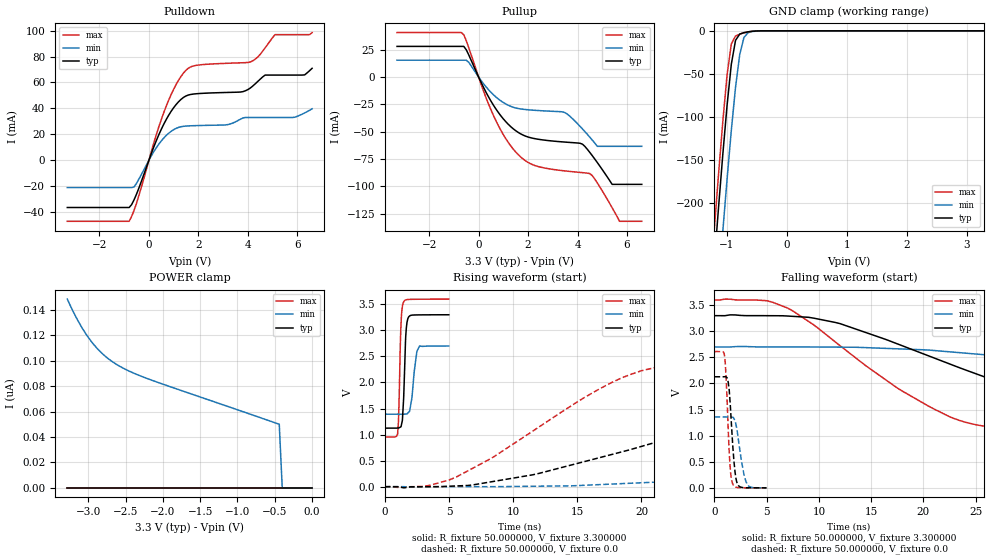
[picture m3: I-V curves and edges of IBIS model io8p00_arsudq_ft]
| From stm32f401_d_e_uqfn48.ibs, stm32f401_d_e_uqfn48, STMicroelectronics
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|   Model io8p00_arsudq_ft
[Model]  io8p00_arsudq_ft
Model_type I/O
Polarity   Non-Inverting
Enable   Active-Low
Vinl =   0.990000V
Vinh =   2.310000V
Vmeas =  1.650000V
Cref =   50.000000pF
Rref =   100.000000M
Vref =   0.0V
C_comp   2.292100pF   2.228000pF   2.366600pF
[Temperature Range]   25.000000   0.125000k   -40.000000
[Pullup Reference]   3.300000V   2.700000V   3.600000V
[Pulldown Reference]   0.0V   0.0V   0.0V
[POWER Clamp Reference]   3.300000V   2.700000V   3.600000V
[GND Clamp Reference]   0.0V   0.0V   0.0V
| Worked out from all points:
|   slope of the pulldown table from 0 to 0.495 V, typ, clamps not added: 20.9 ohm
|   slope of the pullup table from 0 to 0.495 V, typ, clamps not added: 22.6 ohm
|   GND clamp passes 1 mA (typ) near -0.62 V on its own axis
|   rising waveform, R_fixture 50.000000, V_fixture 3.300000: 20-80 % time 190ps typ, 338ps min, 164ps max; typ from 1.12 V to 3.3 V
|   rising waveform, R_fixture 50.000000, V_fixture 0.0: 20-80 % time 19.7ns typ, 51ns min, 10.3ns max; typ from 0 V to 2.13 V
|   falling waveform, R_fixture 50.000000, V_fixture 3.300000: 20-80 % time 18.6ns typ, 39.1ns min, 11.5ns max; typ from 3.3 V to 1.12 V
|   falling waveform, R_fixture 50.000000, V_fixture 0.0: 20-80 % time 434ps typ, 633ps min, 343ps max; typ from 2.13 V to 0 V
[Pulldown]
|Voltage   I(typ)   I(min)   I(max)
-3.3V     -36.46mA   -21.09mA   -47.09mA
-800mV    -36.46mA   -21.09mA   -47.09mA
-600mV    -30.5mA    -20.54mA   -38.69mA
700mV     31.4mA     19.11mA    41.71mA
1.2V      45.15mA    25.37mA    61.75mA
1.6V      50.35mA    26.5mA     71.06mA
3.1V      52.28mA    27.26mA    74.76mA
4.1V      55.7mA     32.99mA    75.81mA
4.7V      65.72mA    32.99mA    86.7mA
5.1V      65.72mA    32.99mA    96.91mA
6.3V      65.88mA    36.51mA    96.91mA
6.6V      70.94mA    39.72mA    98.51mA
[Pullup]
|Voltage   I(typ)   I(min)   I(max)
-3.3V     28.04mA    15.43mA    40.69mA
-700mV    28.04mA    15.43mA    40.69mA
-400mV    20.31mA    13.47mA    26.93mA
600mV     -25.77mA   -16.23mA   -35.14mA
1.6V      -50.64mA   -28.81mA   -70.96mA
3.5V      -59.53mA   -32.65mA   -85.92mA
4.2V      -61.43mA   -47.48mA   -87.46mA
4.5V      -69.07mA   -55.12mA   -88.38mA
4.8V      -78.22mA   -63.4mA    -96.83mA
5.4V      -98.2mA    -63.4mA    -119.6mA
5.7V      -98.2mA    -63.4mA    -132mA
6.6V      -98.2mA    -63.4mA    -132mA
[GND_clamp]
|Voltage   I(typ)   I(min)   I(max)
-3.3V     -2.319A    -2.398A    -2.292A
-1.2V     -265.5mA   -356.1mA   -227.2mA
-1.13V    -202.6mA   -292.9mA   -164.1mA
-1.06V    -142.2mA   -231.2mA   -104.1mA
-990mV    -85.98mA   -171.6mA   -50.72mA
-920mV    -38.8mA    -115.5mA   -15.28mA
-850mV    -11.08mA   -65.6mA    -6.001mA
-780mV    -3.782mA   -27.42mA   -3.876mA
-710mV    -2.086mA   -7.69mA    -2.381mA
-640mV    -1.147mA   -2.118mA   -1.22mA
-570mV    -523.9uA   -798.4uA   -476.8uA
3.28V     0A         0A         0A
[POWER_clamp]
|Voltage   I(typ)   I(min)   I(max)
-3.28V    0A         148.5nA    0A
-3.2V     0A         138.6nA    0A
-3.12V    0A         129.7nA    0A
-3.04V    0A         122nA      0A
-2.96V    0A         115.3nA    0A
-2.8V     0A         105.1nA    0A
-2.6V     0A         96.44nA    0A
-2.4V     0A         90.52nA    0A
-2.16V    0A         84.97nA    0A
-440mV    0A         50.04nA    0A
-400mV    0A         0A         0A
0V        0A         0A         0A
[Ramp]
| variable   typ   min   max
dV/dt_r  1.27740/19.68906n   0.81540/50.98348n   1.56732/10.32996n
dV/dt_f  1.30734/18.58362n   0.78450/39.11759n   1.58789/11.43308n
R_load = 50.000000
[Rising Waveform]
R_fixture= 50.000000
V_fixture= 3.300000
V_fixture_min= 2.700000
V_fixture_max= 3.600000
|time   V(typ)   V(min)   V(max)
0s        1.124V     1.392V     953.5mV
1.001ns   1.126V     1.392V     1.018V
1.071ns   1.128V     1.392V     1.288V
1.251ns   1.149V     1.392V     3.035V
1.461ns   1.66V      1.391V     3.543V
1.632ns   2.882V     1.394V     3.586V
1.862ns   3.259V     1.43V      3.594V
2.503ns   3.297V     2.597V     3.597V
2.703ns   3.297V     2.698V     3.598V
4.985ns   3.3V       2.7V       3.6V
[Rising Waveform]
R_fixture= 50.000000
V_fixture= 0.0
V_fixture_min= 0.0
V_fixture_max= 0.0
|time   V(typ)   V(min)   V(max)
0s        4.932nV    245.7nV    3.133nV
5.506ns   13.81mV    -141.5uV   177.7mV
11.51ns   227.5mV    8.254mV    1.064V
19.02ns   703.8mV    64.87mV    2.142V
27.53ns   1.299V     163.4mV    2.488V
38.54ns   1.854V     360.2mV    2.577V
57.56ns   2.068V     710.1mV    2.608V
89.09ns   2.119V     1.139V     2.612V
117.6ns   2.128V     1.298V     2.612V
249.2ns   2.129V     1.359V     2.612V
[Falling Waveform]
R_fixture= 50.000000
V_fixture= 3.300000
V_fixture_min= 2.700000
V_fixture_max= 3.600000
|time   V(typ)   V(min)   V(max)
0s        3.3V       2.7V       3.6V
5.506ns   3.299V     2.7V       3.561V
12.01ns   3.148V     2.696V     2.726V
22.52ns   2.374V     2.607V     1.362V
31.53ns   1.733V     2.433V     1.074V
37.54ns   1.446V     2.289V     1.03V
46.55ns   1.275V     2.066V     998mV
62.56ns   1.186V     1.74V      969.9mV
86.09ns   1.145V     1.529V     956.6mV
249.2ns   1.124V     1.392V     953.5mV
[Falling Waveform]
R_fixture= 50.000000
V_fixture= 0.0
V_fixture_min= 0.0
V_fixture_max= 0.0
|time   V(typ)   V(min)   V(max)
0s        2.129V     1.359V     2.612V
981ps     2.13V      1.359V     2.507V
1.151ns   2.12V      1.358V     1.947V
1.411ns   1.87V      1.359V     686.9mV
1.542ns   1.49V      1.361V     297.7mV
1.742ns   832.6mV    1.354V     78.17mV
2.152ns   100.6mV    1.12V      8.582mV
2.833ns   4.24mV     245.4mV    1.262mV
3.123ns   1.695mV    72.93mV    990.4uV
4.985ns   4.932nV    245.7nV    3.133nV
